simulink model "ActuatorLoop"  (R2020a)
settings: Solver=FixedStepDiscrete  StartTime=0.0  StopTime=10.0  FixedStep=0.001  RelTol=1e-3  EnableMultiTasking=on
model workspace (MAT data in the model file):
  Kd : Simulink.Parameter (value not decoded)
  Ki : Simulink.Parameter (value not decoded)
  Kp : Simulink.Parameter (value not decoded)
  Ts : Simulink.Parameter (value not decoded)
symbols that are objects in the model workspace (value not decoded): Kd, Ki, Kp, Ts
undefined symbols (not defined in the file or in its folder): DiscIntNeverNeededParam
libraries: simulink x2

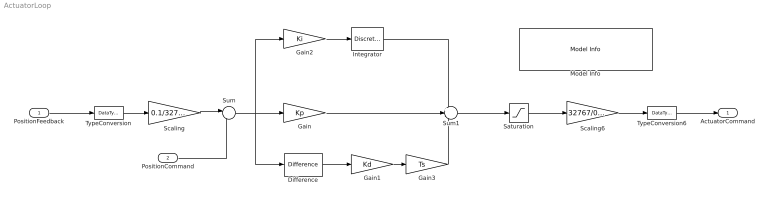
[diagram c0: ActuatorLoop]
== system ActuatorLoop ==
  PositionFeedback : Inport  RequirementInfo={} %GIDa_7cfb5098_cfb3_4ea3_a772_b110fc5247af  OutMin=-32768  OutMax=32767  OutDataTypeStr=int16  PortDimensions=1  SampleTime=0.001
  PositionCommand : Inport  RequirementInfo={} %GIDa_6af42174_6d82_4ebc_8bab_c19e6798c116  Port=2  OutMin=-0.1  OutMax=0.1  OutDataTypeStr=double  PortDimensions=1  SampleTime=0.001
  Difference : simulink/Discrete/Difference  RequirementInfo={} %GIDa_90d6b033_9cb9_40c7_b35e_033491e477c9  ICPrevInput=0.0  OutMin=[]  OutMax=[]  OutDataType=fixdt(1, 16)  OutScaling=2^-10  DoSatur=off
  Gain : Gain  RequirementInfo={} %GIDa_81261c78_7d90_4c3c_8a54_887bf05a630d  Gain=Kp
  Gain1 : Gain  RequirementInfo={} %GIDa_5d7d8362_1967_4992_bb3b_38a72ebc61ca  Gain=Kd
  Gain2 : Gain  RequirementInfo={} %GIDa_1c3736c2_de3f_4491_b8cf_7dd8c6c6f71b  Gain=Ki
  Gain3 : Gain  RequirementInfo={} %GIDa_5d7d8362_1967_4992_bb3b_38a72ebc61ca  Gain=Ts
  Integrator : DiscreteIntegrator  RequirementInfo={} %GIDa_aa124dc7_6443_4cbb_bb02_1cdd6b45c090  SampleTime=-1  LimitOutput=on  UpperSaturationLimit=0.1  LowerSaturationLimit=-0.1  ICPrevOutput=DiscIntNeverNeededParam  ICPrevScaledInput=DiscIntNeverNeededParam
  Model Info : simulink/Model-Wide Utilities/Model Info  Frame=on  DisplayStringWithTags=|  HorizontalTextAlignment=Center  LeftAlignmentValue=0.5
      | Model Name: %<ModelName>
      | Model Version: %<ModelVersion>
      | Last Modified: %<LastModificationDate>
      | 
      | Copyright 2016 The MathWorks, Inc.
  Saturation : Saturate  RequirementInfo={} %GIDa_8ac92945_a301_4fef_a0ea_5ecfd6c47c62  UpperLimit=0.3  LowerLimit=-0.3
  Scaling : Gain  Gain=0.1/32767
  Scaling6 : Gain  Gain=32767/0.3  SaturateOnIntegerOverflow=on
  Sum : Sum  RequirementInfo={} %GIDa_d38775e8_f124_43a8_82cc_6598fe8ea0e4  Inputs=|-+
  Sum1 : Sum  RequirementInfo={} %GIDa_c0b02d8e_6114_4add_ae74_a5491d42d294  Inputs=++-
  TypeConversion : DataTypeConversion  OutDataTypeStr=double
  TypeConversion6 : DataTypeConversion  OutDataTypeStr=int16
  ActuatorCommand : Outport  RequirementInfo={} %GIDa_d1666590_09eb_4dbd_9180_483dbf5dbc22  VectorParamsAs1DForOutWhenUnconnected=off
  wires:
  PositionCommand/1 -> Sum/2
  Sum/1 -> Difference/1, Gain2/1, Gain/1
  Gain/1 -> Sum1/2
  Sum1/1 -> Saturation/1
  Integrator/1 -> Sum1/1
  Difference/1 -> Gain1/1
  Gain1/1 -> Gain3/1
  Gain2/1 -> Integrator/1
  PositionFeedback/1 -> TypeConversion/1
  TypeConversion/1 -> Scaling/1
  Scaling/1 -> Sum/1
  Scaling6/1 -> TypeConversion6/1
  Saturation/1 -> Scaling6/1
  TypeConversion6/1 -> ActuatorCommand/1
  Gain3/1 -> Sum1/3
